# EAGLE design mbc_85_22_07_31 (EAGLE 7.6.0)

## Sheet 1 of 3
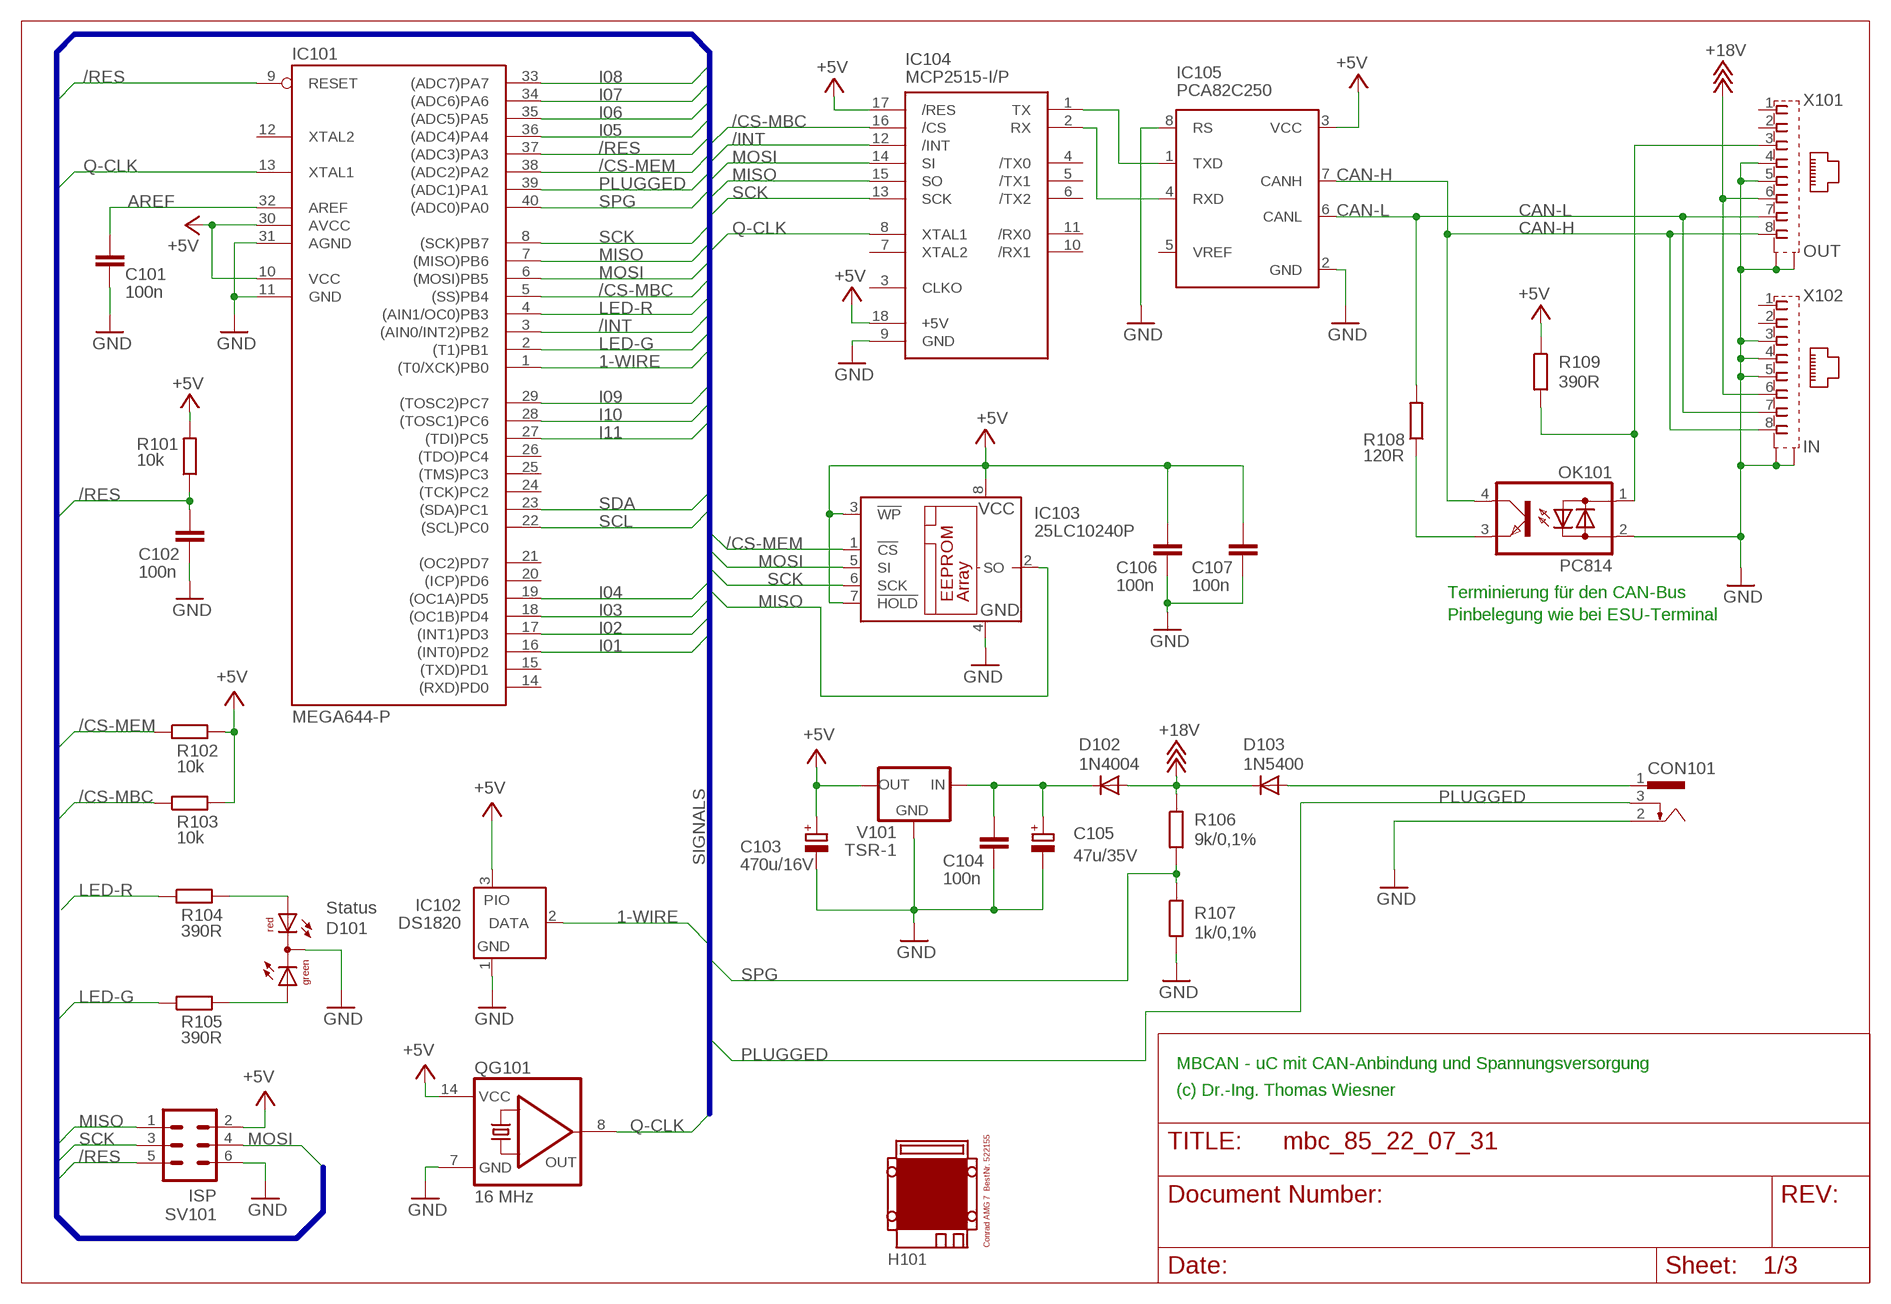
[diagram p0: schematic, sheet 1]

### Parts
C101  100n  C-EU025-025X050  [C025-025X050]
C102  100n  C-EU025-025X050  [C025-025X050]
C103  470u/16V  CPOL-EUE3.5-8  [E3,5-8]
C104  100n  C-EU025-025X050  [C025-025X050]
C105  47u/35V  CPOL-EUE2.5-7  [E2,5-7]
C106  100n  C-EU025-025X050  [C025-025X050]
C107  100n  C-EU025-025X050  [C025-025X050]
CON101  POWER-JACK  [POWER-JACK]
D101  Status  DUOLED5MM  [DUOLED5MM]
D102  1N4004  [DO41-10]
D103  1N5400  [DO201-15]
H101  MODULGEHÄUSE-AMG-7  [MODULGEHÄUSE-AMG-7]
IC101  MEGA644-P  MEGA323-P  [DIL40]
IC102  DS1820  DS2405  [TO92-]
IC103  25LC10240P  25LC040P  [DIL8]
IC104  MCP2515-I/P  MCP2510-I/P  [DIL18]
IC105  PCA82C250  [DIL08]
OK101  PC814  [DIL04]
QG101  16 MHz  QG5860  [DIL14S]
R101  10k  R-EU_0207/10  [0207/10]
R102  10k  R-EU_0207/10  [0207/10]
R103  10k  R-EU_0207/10  [0207/10]
R104  390R  R-EU_0207/10  [0207/10]
R105  390R  R-EU_0207/10  [0207/10]
R106  9k/0,1%  R-EU_0207/10  [0207/10]
R107  1k/0,1%  R-EU_0207/10  [0207/10]
R108  120R  R-EU_0207/10  [0207/10]
R109  390R  R-EU_0207/10  [0207/10]
SV101  ISP  ML6  [ML6]
V101  TSR-1  [TRACO-TSR-1]
X101  OUT  0446200002  [0446200002]
X102  IN  0446200002  [0446200002]

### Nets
1-WIRE: IC101.1((T0/XCK)PB0) IC102.2(DATA)
+5V: C103.+ C106.1 C107.1 IC101.10(VCC) IC101.30(AVCC) IC102.3(PIO) IC103.3(!WP) IC103.7(!HOLD) IC103.8(VCC) IC104.17(/RES) IC104.18(+5V) IC105.3(VCC) QG101.14(VCC) R101.2 R102.2 R103.2 R109.1 SV101.2 V101.OUT ; also sheet 2
+18V: D102.A D103.C R106.1 X101.6 X102.6
/CS-MBC: IC101.5((SS)PB4) IC104.16(/CS) R103.1
/CS-MEM: IC101.38((ADC2)PA2) IC103.1(!CS) R102.1
/INT: IC101.3((AIN0/INT2)PB2) IC104.12(/INT)
/RES: C102.1 IC101.9(RESET) IC101.37((ADC3)PA3) R101.1 SV101.5
AREF: C101.1 IC101.32(AREF)
CAN-H: IC105.7(CANH) OK101.4(C) X101.8 X102.8
CAN-L: IC105.6(CANL) R108.2 X101.7 X102.7
GND: C101.2 C102.2 C103.- C104.2 C105.- C106.2 C107.2 CON101.2 D101.K(C) IC101.11(GND) IC101.31(AGND) IC102.1(GND) IC103.4(GND) IC104.9(GND) IC105.2(GND) IC105.8(RS) OK101.2(AC2) QG101.7(GND) R107.2 SV101.6 V101.GND X101.4 X101.5 X101.S@1(S1) X101.S@2(S2) X102.3 X102.4 X102.5 X102.S@1(S1) X102.S@2(S2) ; also sheet 2
I01: IC101.16((INT0)PD2) ; also sheet 2
I02: IC101.17((INT1)PD3) ; also sheet 2
I03: IC101.18((OC1B)PD4) ; also sheet 2
I04: IC101.19((OC1A)PD5) ; also sheet 2
I05: IC101.36((ADC4)PA4) ; also sheet 2
I06: IC101.35((ADC5)PA5) ; also sheet 2
I07: IC101.34((ADC6)PA6) ; also sheet 2
I08: IC101.33((ADC7)PA7) ; also sheet 2
I09: IC101.29((TOSC2)PC7) ; also sheet 2
I10: IC101.28((TOSC1)PC6) ; also sheet 2
I11: IC101.27((TDI)PC5) ; also sheet 2
LED-G: IC101.2((T1)PB1) R105.1
LED-R: IC101.4((AIN1/OC0)PB3) R104.1
MISO: IC101.7((MISO)PB6) IC103.2(SO) IC104.15(SO) SV101.1
MOSI: IC101.6((MOSI)PB5) IC103.5(SI) IC104.14(SI) SV101.4
N$1: IC104.1(TX) IC105.1(TXD)
N$2: IC104.2(RX) IC105.4(RXD)
N$4: OK101.3(E) R108.1
N$6: C104.1 C105.+ D102.C V101.IN
N$7: OK101.1(AC1) R109.2 X101.3
N$9: D101.AR R104.2
N$13: D101.AG R105.2
PLUGGED: CON101.3 IC101.39((ADC1)PA1)
Q-CLK: IC101.13(XTAL1) IC104.8(XTAL1) QG101.8(OUT)
SCK: IC101.8((SCK)PB7) IC103.6(SCK) IC104.13(SCK) SV101.3
SCL: IC101.22((SCL)PC0) ; also sheet 2
SDA: IC101.23((SDA)PC1) ; also sheet 2
SPG: IC101.40((ADC0)PA0) R106.2 R107.1
V-NETZTEIL1: CON101.1 D103.A
Unconnected: IC101.12(XTAL2) IC101.14((RXD)PD0) IC101.15((TXD)PD1) IC101.20((ICP)PD6) IC101.21((OC2)PD7) IC101.24((TCK)PC2) IC101.25((TMS)PC3) IC101.26((TDO)PC4) IC104.3(CLKO) IC104.4(/TX0) IC104.5(/TX1) IC104.6(/TX2) IC104.7(XTAL2) IC104.10(/RX1) IC104.11(/RX0) IC105.5(VREF) X101.1 X101.2 X102.1 X102.2

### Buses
SIGNALS

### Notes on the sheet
- Terminierung für den CAN-Bus
- Pinbelegung wie bei ESU-Terminal
- MBCAN - uC mit CAN-Anbindung und Spannungsversorgung
- (c) Dr.-Ing. Thomas Wiesner

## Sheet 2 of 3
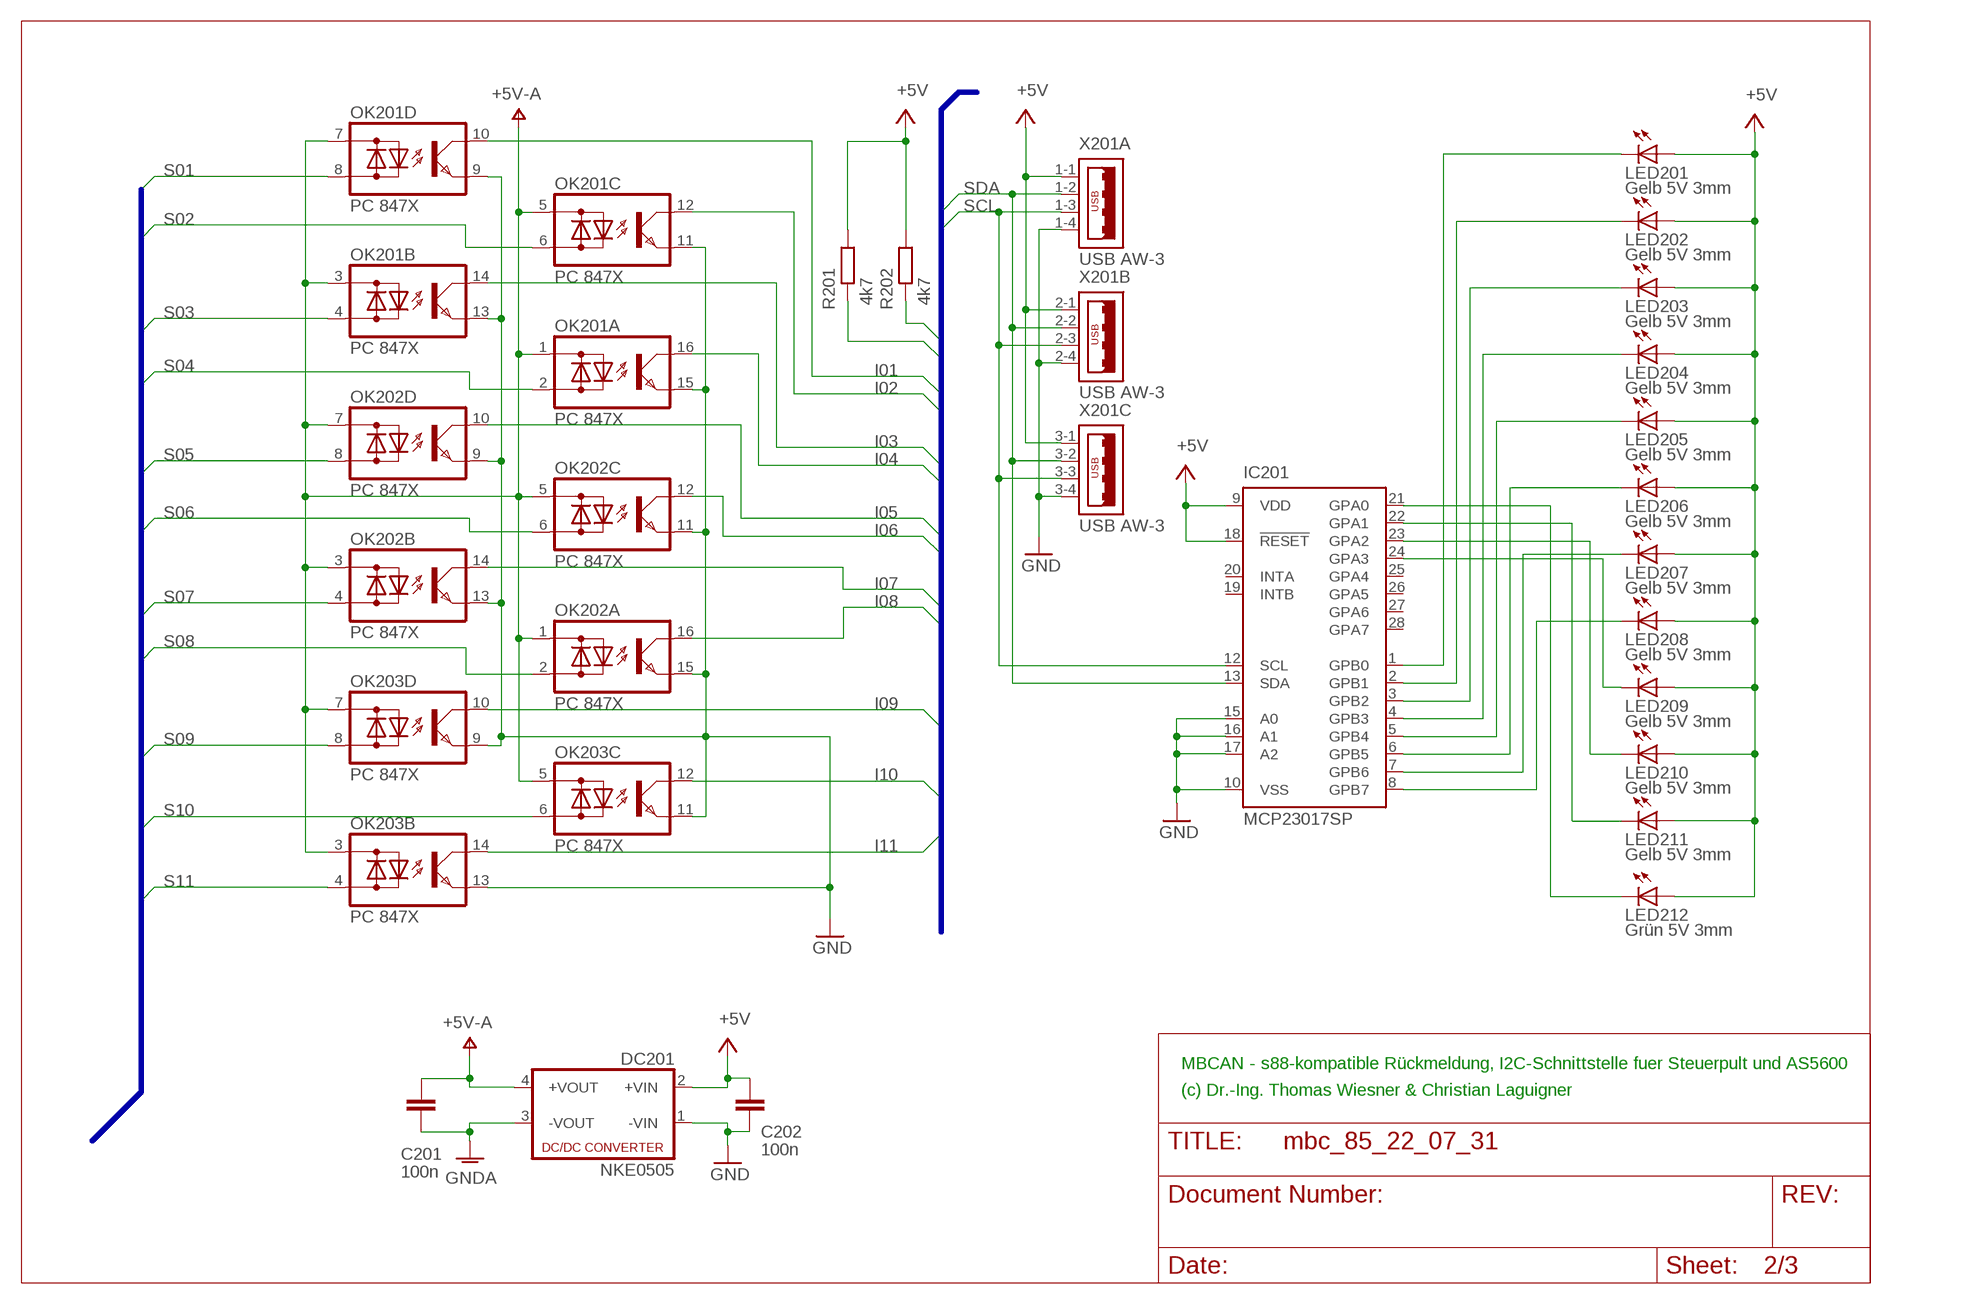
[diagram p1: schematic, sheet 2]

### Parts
C201  100n  C-EU025-025X050  [C025-025X050]
C202  100n  C-EU025-025X050  [C025-025X050]
DC201  NKE0505  NME  [NME]
IC201  MCP23017SP  [DIL28-3]
LED201  Gelb 5V 3mm  LED3MM  [LED3MM]
LED202  Gelb 5V 3mm  LED3MM  [LED3MM]
LED203  Gelb 5V 3mm  LED3MM  [LED3MM]
LED204  Gelb 5V 3mm  LED3MM  [LED3MM]
LED205  Gelb 5V 3mm  LED3MM  [LED3MM]
LED206  Gelb 5V 3mm  LED3MM  [LED3MM]
LED207  Gelb 5V 3mm  LED3MM  [LED3MM]
LED208  Gelb 5V 3mm  LED3MM  [LED3MM]
LED209  Gelb 5V 3mm  LED3MM  [LED3MM]
LED210  Gelb 5V 3mm  LED3MM  [LED3MM]
LED211  Gelb 5V 3mm  LED3MM  [LED3MM]
LED212  Grün 5V 3mm  LED3MM  [LED3MM]
OK201  PC 847X  TIL196  [DIL16]
OK202  PC 847X  TIL196  [DIL16]
OK203  PC 847X  TIL196  [DIL16]
R201  4k7  R-EU_0207/10  [0207/10]
R202  4k7  R-EU_0207/10  [0207/10]
X201  USB AW-3  USB_3P-85-32003-00X-1  [85-32003-00X-1]

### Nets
+5V: C202.1 DC201.2(+VIN) IC201.9(VDD) IC201.18(!RESET) LED201.A LED202.A LED203.A LED204.A LED205.A LED206.A LED207.A LED208.A LED209.A LED210.A LED211.A LED212.A R201.2 R202.2 X201.1-1 X201.2-1 X201.3-1 ; also sheet 1
GND: C202.2 DC201.1(-VIN) IC201.10(VSS) IC201.15(A0) IC201.16(A1) IC201.17(A2) OK201.9(D:E) OK201.11(C:E) OK201.13(B:E) OK201.15(A:E) OK202.9(D:E) OK202.11(C:E) OK202.13(B:E) OK202.15(A:E) OK203.9(D:E) OK203.11(C:E) OK203.13(B:E) X201.1-4 X201.2-4 X201.3-4 ; also sheet 1
GNDA: C201.2 DC201.3(-VOUT) ; also sheet 3
I01: OK201.10(D:C) ; also sheet 1
I02: OK201.12(C:C) ; also sheet 1
I03: OK201.14(B:C) ; also sheet 1
I04: OK201.16(A:C) ; also sheet 1
I05: OK202.10(D:C) ; also sheet 1
I06: OK202.12(C:C) ; also sheet 1
I07: OK202.14(B:C) ; also sheet 1
I08: OK202.16(A:C) ; also sheet 1
I09: OK203.10(D:C) ; also sheet 1
I10: OK203.12(C:C) ; also sheet 1
I11: OK203.14(B:C) ; also sheet 1
N$10: IC201.1(GPB0) LED201.K(C)
N$11: IC201.24(GPA3) LED209.K(C)
N$16: IC201.21(GPA0) LED212.K(C)
N$18: IC201.2(GPB1) LED202.K(C)
N$19: IC201.3(GPB2) LED203.K(C)
N$22: IC201.4(GPB3) LED204.K(C)
N$23: IC201.5(GPB4) LED205.K(C)
N$32: IC201.6(GPB5) LED206.K(C)
N$34: IC201.7(GPB6) LED207.K(C)
N$35: IC201.8(GPB7) LED208.K(C)
N$36: IC201.22(GPA1) LED211.K(C)
N$37: IC201.23(GPA2) LED210.K(C)
S01: OK201.8(D:AC2) ; also sheet 3
S02: OK201.6(C:AC2) ; also sheet 3
S03: OK201.4(B:AC2) ; also sheet 3
S04: OK201.2(A:AC2) ; also sheet 3
S05: OK202.8(D:AC2) ; also sheet 3
S06: OK202.6(C:AC2) ; also sheet 3
S07: OK202.4(B:AC2) ; also sheet 3
S08: OK202.2(A:AC2) ; also sheet 3
S09: OK203.8(D:AC2) ; also sheet 3
S10: OK203.6(C:AC2) ; also sheet 3
S11: OK203.4(B:AC2) ; also sheet 3
SCL: IC201.12(SCL) R201.1 X201.1-3 X201.2-3 X201.3-3 ; also sheet 1
SDA: IC201.13(SDA) R202.1 X201.1-2 X201.2-2 X201.3-2 ; also sheet 1
V+: C201.1 DC201.4(+VOUT) OK201.1(A:AC1) OK201.3(B:AC1) OK201.5(C:AC1) OK201.7(D:AC1) OK202.1(A:AC1) OK202.3(B:AC1) OK202.5(C:AC1) OK202.7(D:AC1) OK203.3(B:AC1) OK203.5(C:AC1) OK203.7(D:AC1) ; supply symbol labelled +5V-A
Unconnected: IC201.19(INTB) IC201.20(INTA) IC201.25(GPA4) IC201.26(GPA5) IC201.27(GPA6) IC201.28(GPA7) OK203.1(A:AC1) OK203.2(A:AC2) OK203.15(A:E) OK203.16(A:C)

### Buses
B$1
B$2

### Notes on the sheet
- MBCAN - s88-kompatible Rückmeldung, I2C-Schnittstelle fuer Steuerpult und AS5600
- (c) Dr.-Ing. Thomas Wiesner & Christian Laguigner

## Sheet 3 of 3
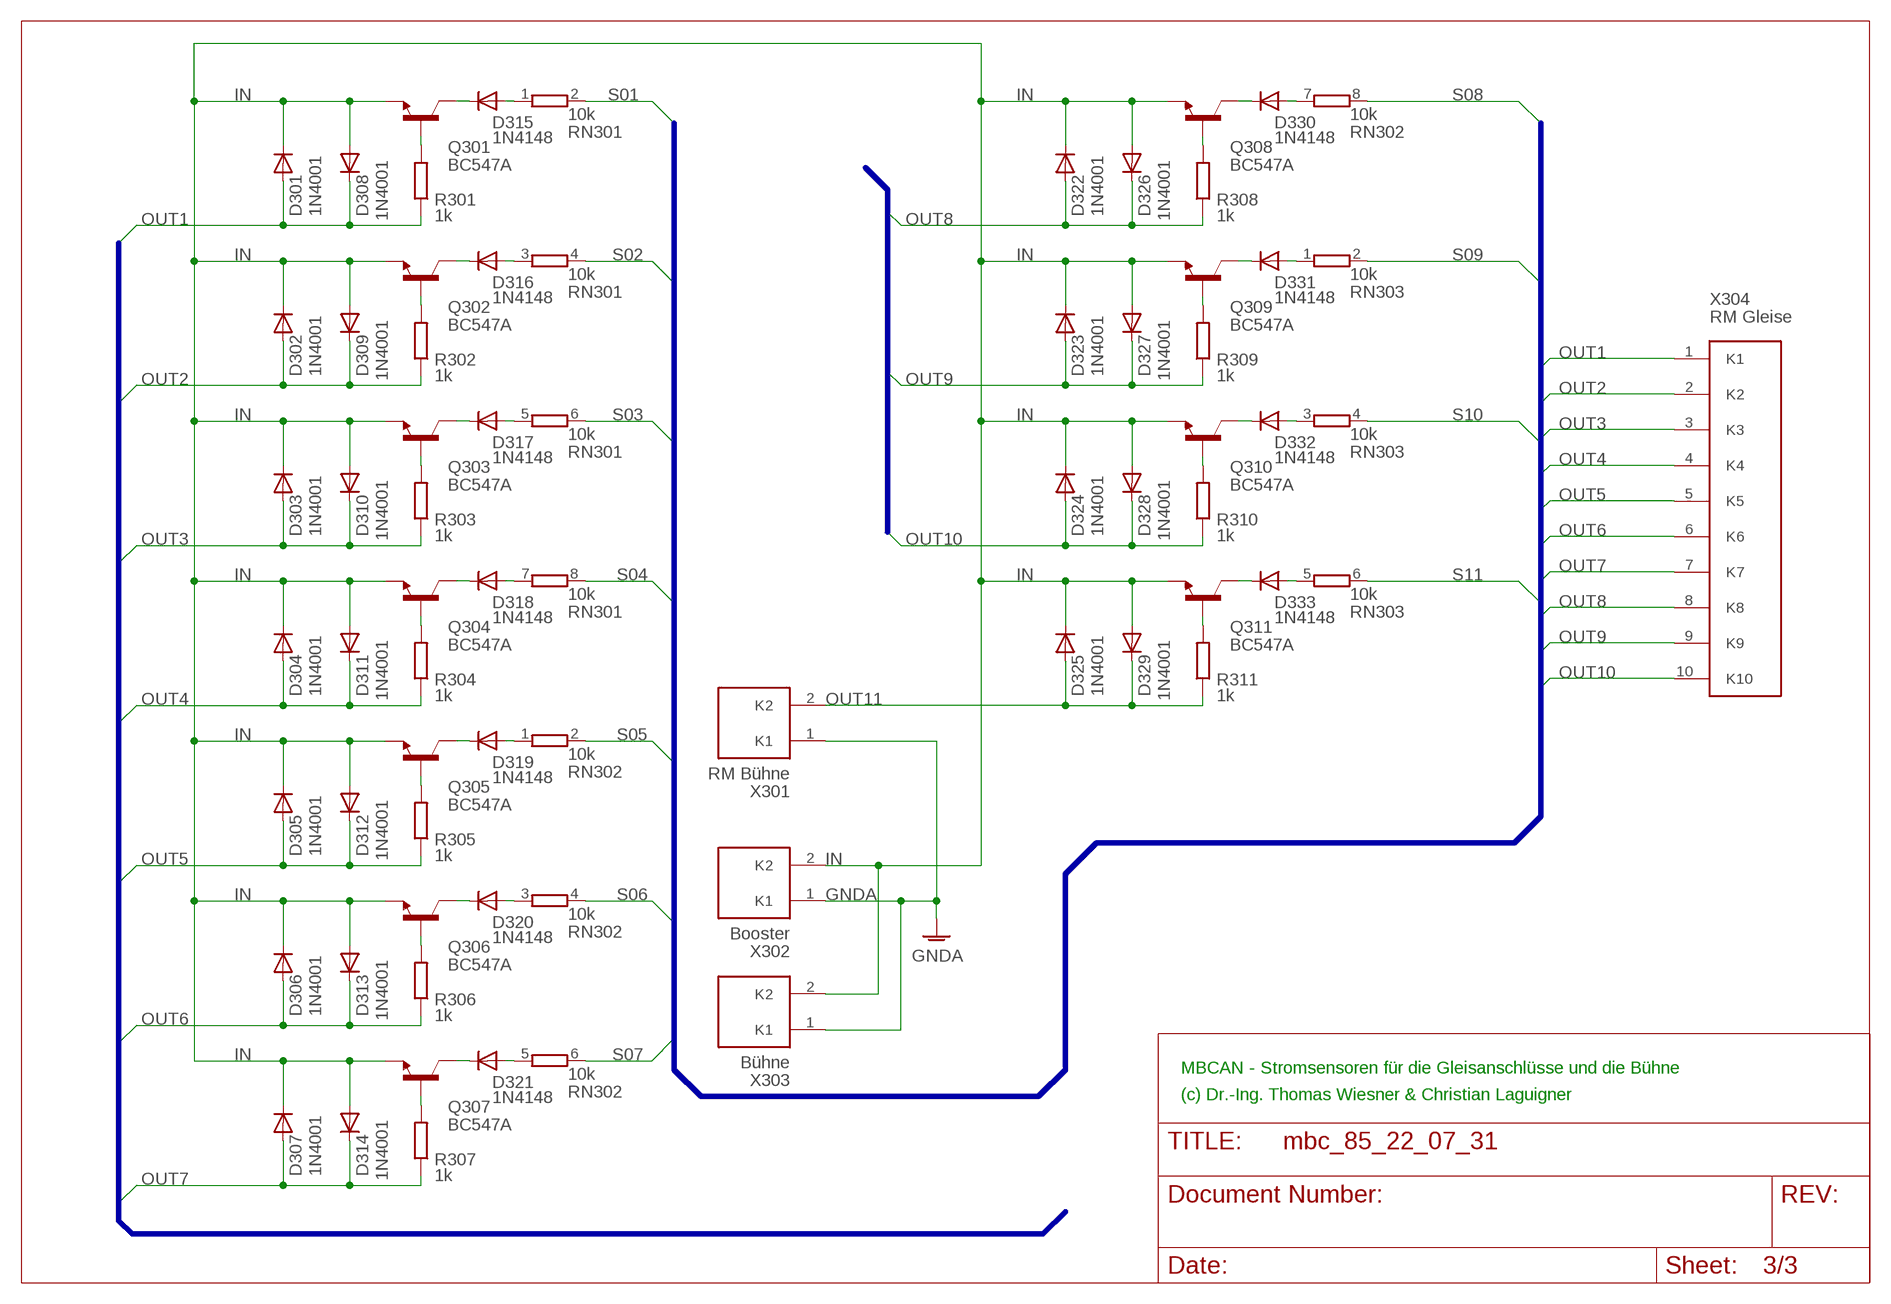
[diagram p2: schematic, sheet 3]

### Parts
D301  1N4001  1N4004  [DO41-10]
D302  1N4001  1N4004  [DO41-10]
D303  1N4001  1N4004  [DO41-10]
D304  1N4001  1N4004  [DO41-10]
D305  1N4001  1N4004  [DO41-10]
D306  1N4001  1N4004  [DO41-10]
D307  1N4001  1N4004  [DO41-10]
D308  1N4001  1N4004  [DO41-10]
D309  1N4001  1N4004  [DO41-10]
D310  1N4001  1N4004  [DO41-10]
D311  1N4001  1N4004  [DO41-10]
D312  1N4001  1N4004  [DO41-10]
D313  1N4001  1N4004  [DO41-10]
D314  1N4001  1N4004  [DO41-10]
D315  1N4148  1N4148DO35-10  [DO35-10]
D316  1N4148  1N4148DO35-10  [DO35-10]
D317  1N4148  1N4148DO35-10  [DO35-10]
D318  1N4148  1N4148DO35-10  [DO35-10]
D319  1N4148  1N4148DO35-10  [DO35-10]
D320  1N4148  1N4148DO35-10  [DO35-10]
D321  1N4148  1N4148DO35-10  [DO35-10]
D322  1N4001  1N4004  [DO41-10]
D323  1N4001  1N4004  [DO41-10]
D324  1N4001  1N4004  [DO41-10]
D325  1N4001  1N4004  [DO41-10]
D326  1N4001  1N4004  [DO41-10]
D327  1N4001  1N4004  [DO41-10]
D328  1N4001  1N4004  [DO41-10]
D329  1N4001  1N4004  [DO41-10]
D330  1N4148  1N4148DO35-10  [DO35-10]
D331  1N4148  1N4148DO35-10  [DO35-10]
D332  1N4148  1N4148DO35-10  [DO35-10]
D333  1N4148  1N4148DO35-10  [DO35-10]
Q301  BC547A  [TO92]
Q302  BC547A  [TO92]
Q303  BC547A  [TO92]
Q304  BC547A  [TO92]
Q305  BC547A  [TO92]
Q306  BC547A  [TO92]
Q307  BC547A  [TO92]
Q308  BC547A  [TO92]
Q309  BC547A  [TO92]
Q310  BC547A  [TO92]
Q311  BC547A  [TO92]
R301  1k  R-EU_0207/10  [0207/10]
R302  1k  R-EU_0207/10  [0207/10]
R303  1k  R-EU_0207/10  [0207/10]
R304  1k  R-EU_0207/10  [0207/10]
R305  1k  R-EU_0207/10  [0207/10]
R306  1k  R-EU_0207/10  [0207/10]
R307  1k  R-EU_0207/10  [0207/10]
R308  1k  R-EU_0207/10  [0207/10]
R309  1k  R-EU_0207/10  [0207/10]
R310  1k  R-EU_0207/10  [0207/10]
R311  1k  R-EU_0207/10  [0207/10]
RN301  10k  E4RP  [SIL8]
RN302  10k  E4RP  [SIL8]
RN303  10k  E4RP  [SIL8]
X301  RM Bühne  AKL182-2  [AKL182-2]
X302  Booster  AKL182-2  [AKL182-2]
X303  Bühne  AKL182-2  [AKL182-2]
X304  RM Gleise  AKL182-10  [AKL182-10]

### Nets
GNDA: X301.1(K1) X302.1(K1) X303.1(K1) ; also sheet 2
IN: D301.C D302.C D303.C D304.C D305.C D306.C D307.C D308.A D309.A D310.A D311.A D312.A D313.A D314.A D322.C D323.C D324.C D325.C D326.A D327.A D328.A D329.A Q301.1(E) Q302.1(E) Q303.1(E) Q304.1(E) Q305.1(E) Q306.1(E) Q307.1(E) Q308.1(E) Q309.1(E) Q310.1(E) Q311.1(E) X302.2(K2) X303.2(K2)
N$27: Q301.2(B) R301.2
N$33: D315.C Q301.3(C)
N$38: D315.A RN301.1
N$40: Q302.2(B) R302.2
N$41: D316.C Q302.3(C)
N$49: D316.A RN301.3
N$51: Q303.2(B) R303.2
N$52: D317.C Q303.3(C)
N$53: D317.A RN301.5
N$55: Q304.2(B) R304.2
N$56: D318.C Q304.3(C)
N$57: D318.A RN301.7
N$59: Q305.2(B) R305.2
N$60: D319.C Q305.3(C)
N$61: D319.A RN302.1
N$63: Q306.2(B) R306.2
N$66: D320.C Q306.3(C)
N$67: D320.A RN302.3
N$69: Q307.2(B) R307.2
N$70: D321.C Q307.3(C)
N$71: D321.A RN302.5
N$73: Q308.2(B) R308.2
N$74: D330.C Q308.3(C)
N$75: D330.A RN302.7
N$77: Q309.2(B) R309.2
N$78: D331.C Q309.3(C)
N$79: D331.A RN303.1
N$81: Q310.2(B) R310.2
N$82: D332.C Q310.3(C)
N$83: D332.A RN303.3
N$85: Q311.2(B) R311.2
N$86: D333.C Q311.3(C)
N$87: D333.A RN303.5
OUT1: D301.A D308.C R301.1 X304.1(K1)
OUT2: D302.A D309.C R302.1 X304.2(K2)
OUT3: D303.A D310.C R303.1 X304.3(K3)
OUT4: D304.A D311.C R304.1 X304.4(K4)
OUT5: D305.A D312.C R305.1 X304.5(K5)
OUT6: D306.A D313.C R306.1 X304.6(K6)
OUT7: D307.A D314.C R307.1 X304.7(K7)
OUT8: D322.A D326.C R308.1 X304.8(K8)
OUT9: D323.A D327.C R309.1 X304.9(K9)
OUT10: D324.A D328.C R310.1 X304.10(K10)
OUT11: D325.A D329.C R311.1 X301.2(K2)
S01: RN301.2 ; also sheet 2
S02: RN301.4 ; also sheet 2
S03: RN301.6 ; also sheet 2
S04: RN301.8 ; also sheet 2
S05: RN302.2 ; also sheet 2
S06: RN302.4 ; also sheet 2
S07: RN302.6 ; also sheet 2
S08: RN302.8 ; also sheet 2
S09: RN303.2 ; also sheet 2
S10: RN303.4 ; also sheet 2
S11: RN303.6 ; also sheet 2
Unconnected: RN303.7 RN303.8

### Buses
B$3
B$4
B$5

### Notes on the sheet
- MBCAN - Stromsensoren für die Gleisanschlüsse und die Bühne
- (c) Dr.-Ing. Thomas Wiesner & Christian Laguigner

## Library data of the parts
C101 C102 C104 C106 C107 C201 C202 = rcl:C-EU: CAPACITOR, European symbol
C103 C105 = rcl:CPOL-EU: POLARIZED CAPACITOR, European symbol
CON101 = mbc:POWER-JACK: Power-Stecker für 2,5 mm Hohlbuchse
D101 = led:DUOLED5MM: DUO LED 2 colors, 5 mm, round
D102 D301-D314 D322-D329 = diode:1N4004: DIODE
D103 = diode:1N5400: DIODE
D315-D321 D330-D333 = diode:1N4148: DIODE
DC201 = dc-dc-converter:NME: DC-DC CONVERTER; MF: C & D TECHNOLOGIES, INC; MPN: NME1205D; OC_FARNELL: 1021466; OC_NEWARK: 98B8198
H101 = mbc:MODULGEHÄUSE-AMG-7: Gehäuse
IC101 = atmel:MEGA323-P: MICROCONTROLLER 32 Kbytes FLASH 2 Kbytes SRAM 1 Kbytes EEPROM USART 8-channel 10 bit ADC Source: avr.lbr; OC_FARNELL: unknown; OC_NEWARK: unknown
IC102 = maxim:DS2405: Addressable Switch DALLAS Semiconductor; MF: DALLAS SEMICONDUCTOR; MPN: DS2405; OC_FARNELL: 1188025; OC_NEWARK: 06F4645
IC103 = microchip:25*: Serial EEPROM 4K/ 8K , SPI bus; MF: MICROCHIP; MPN: 25LC040/P; OC_FARNELL: 9758100; OC_NEWARK: 96K4091
IC104 = mbc:MCP2510: BASIC-CAN 2.0a Controller Stand-alone CAN controller von Microchip
IC105 = micro-philips:PCA82C250: CAN CONTROLLER INTERFACE; OC_FARNELL: 3692358; OC_NEWARK: unknown
IC201 = microchip:MCP23017: http://ww1.microchip.com/downloads/en/DeviceDoc/21952a.pdf Source: http://ww1.microchip.com/downloads/en/DeviceDoc/21952a.pdf; MF: MICROCHIP; MPN: MCP23017-E/SP; OC_FARNELL: 1332088; OC_NEWARK: 31K2959
LED201-LED212 = led:LED: LED
OK101 = optocoupler:PC814: SHARP OPTO COUPLER; OC_FARNELL: 9707662; OC_NEWARK: unknown
OK201-OK203 = optocoupler:TIL196: TEXAS INSTRUMENTS OPTO COUPLER; MPN: TIL 196; OC_FARNELL: 1683367; OC_NEWARK: 05R6476
Q301-Q311 = transistor-npn:BC547*: NPN Transistor
QG101 = crystal:QG5860: CRYSTAL RESONATOR; OC_FARNELL: unknown; OC_NEWARK: unknown
R101-R109 R201 R202 R301-R311 = resistor:R-EU_: RESISTOR, European symbol
RN301-RN303 = resistor-sil:E4RP: SIL RESISTOR; OC_FARNELL: unknown; OC_NEWARK: unknown
SV101 = con-ml:ML6: HARTING; OC_FARNELL: unknown; OC_NEWARK: unknown
V101 = mbc:TSR-1: Spannungsregler Hersteller: TRACO Typ: TSR-1 5V: TSR 1-2450 Spg: 5V Strom: 1A Reichelt TSR 1-2450
X101 X102 = mbc:0446200002: RJ-45 INVERTED MODULAR JACK ASSEMBLY WITH RJ-11 KEEPOUT FEATURE Source: Data sheet MOLEX 0446200002 BUCHSE, RJ45, GESCHIRMT Source: Farnell; MF: MOLEX; MPN: 0446200002; OC_FARNELL: 9251910
X201 = con-cypressindustries:USB_3P-: Triple USB Connector Source: www.cypressindustries.com; OC_FARNELL: unknown; OC_NEWARK: unknown
X301-X303 = mbc:AKL182-2: Steckverbinder
X304 = mbc:AKL182-10: Steckverbinder Rastermaß: 3,5 mm Hersteller: RIA Reichelt: Bestellnummer AKL 182-10

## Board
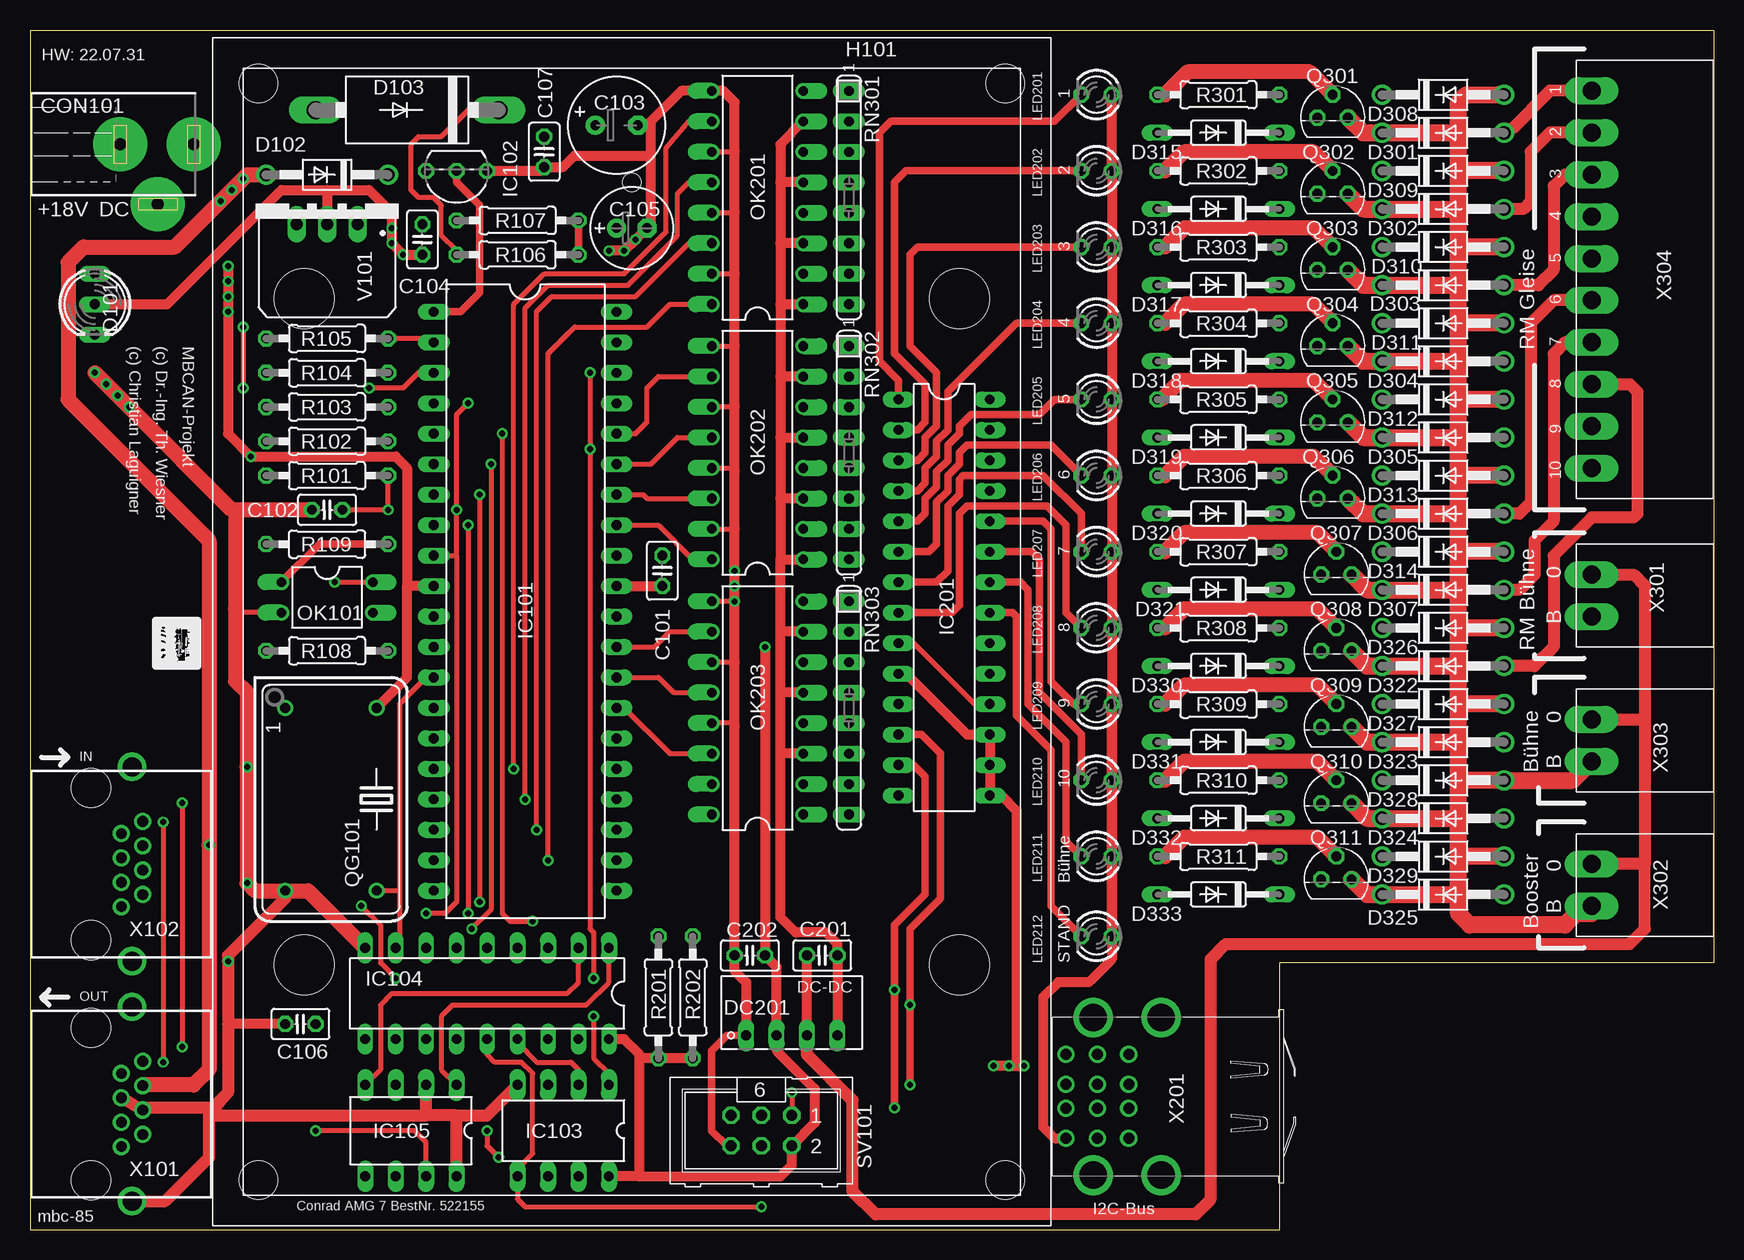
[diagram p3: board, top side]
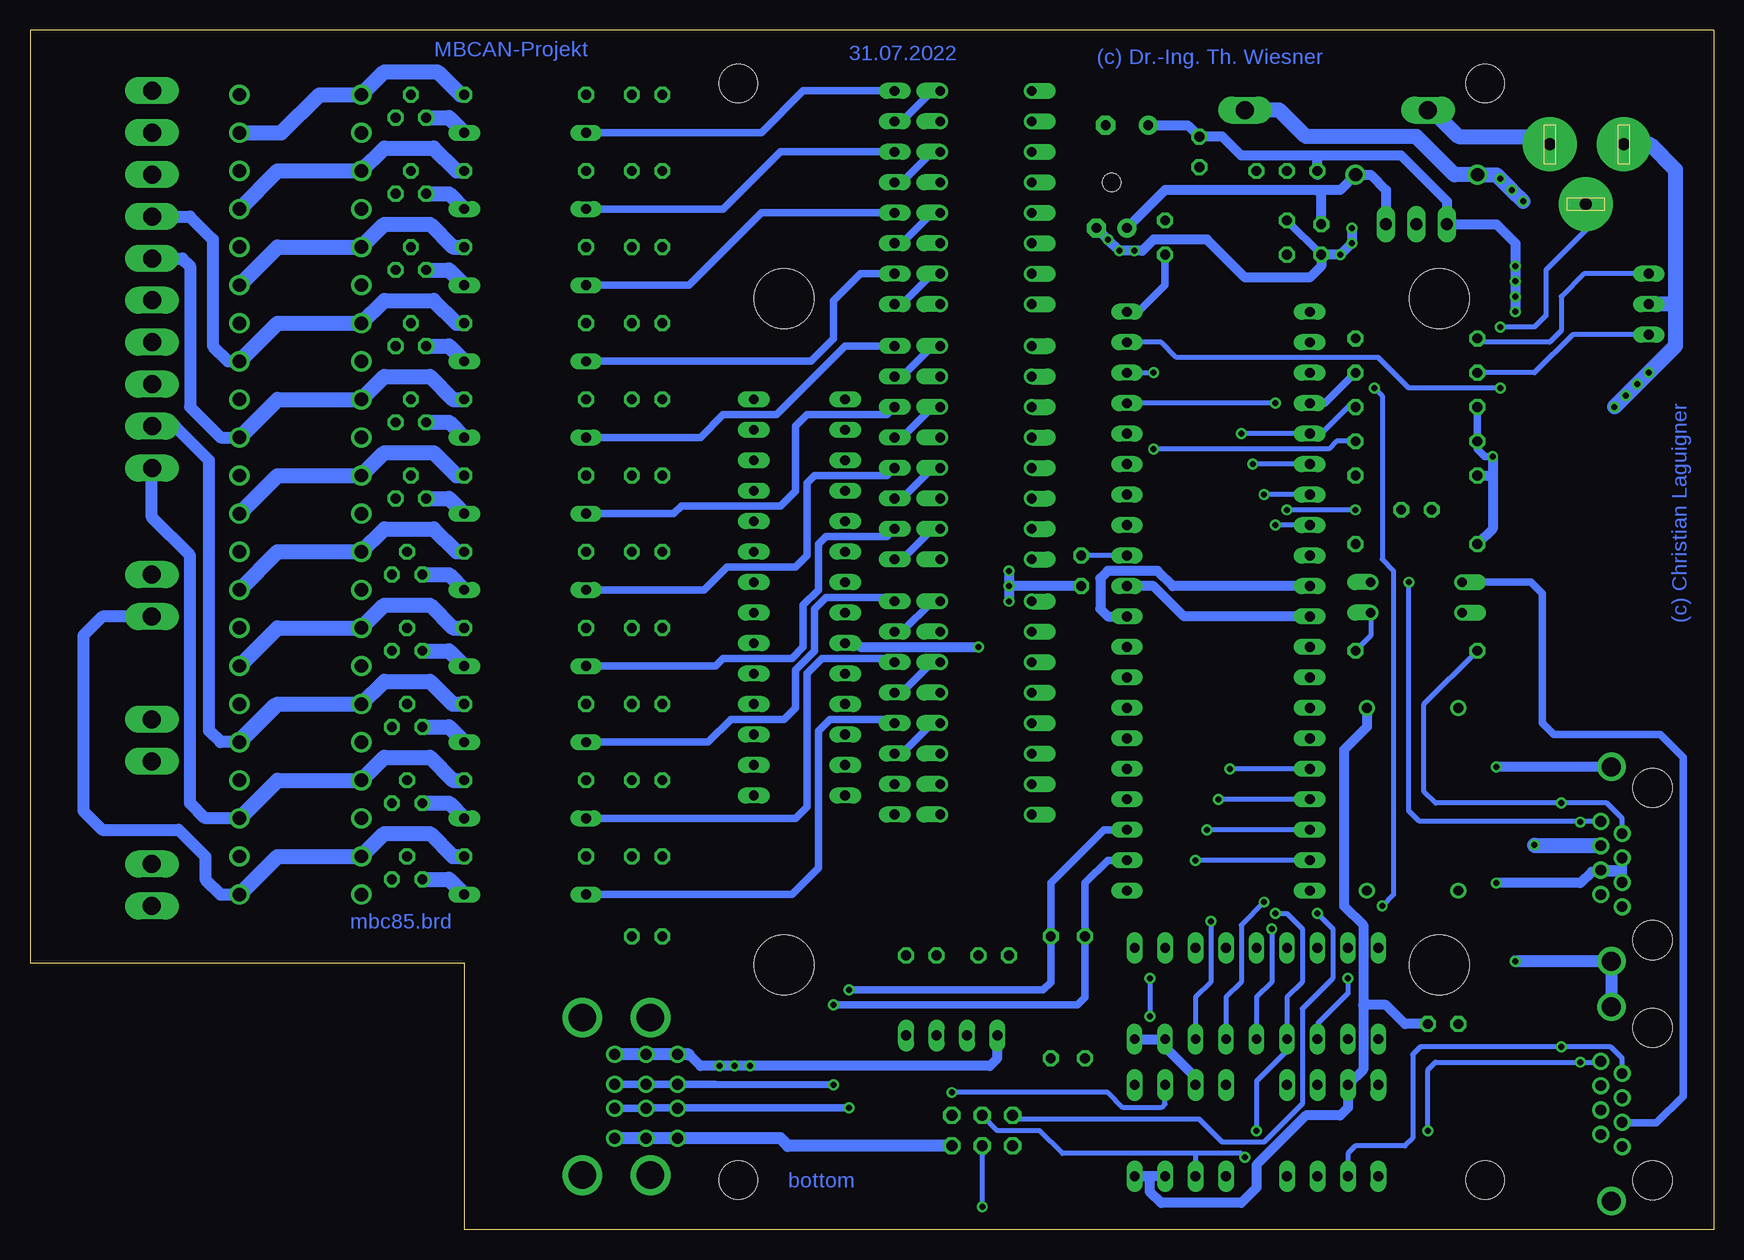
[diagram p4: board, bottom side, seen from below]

Size 140.34 x 100.01 mm. Coordinates in mm from the lower left corner, seen from the top.
Outline: 0,0.02 0,100.01 140.34,100.01 140.34,22.23 104.14,22.23 104.14,0 0,0
Copper layers (1*16): Top 0.035mm / dielectric 1.5mm / Bottom 0.035mm
Design rules "default *": minimum track width 10mil, minimum drill 0.5mm, track to track 8mil, track to pad 8mil, pad to pad 8mil, via to via 8mil, smd to smd 8mil, copper to edge 40mil, drill to drill 8mil, minimum pad ring 10mil, minimum via ring 8mil, stop-mask expansion 4mil, vias tented up to drill 0mil, thermal gap 10mil

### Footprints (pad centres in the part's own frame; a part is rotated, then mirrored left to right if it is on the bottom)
C025-025X050 = drill 0.813 octagon: 1 -1.27,0; 2 1.27,0
E3,5-8 = drill 0.813 pad 1.6: + -1.778,0 | drill 0.813 pad 1.6 octagon: - 1.778,0
E2,5-7 = drill 0.813 pad 1.6: + -1.27,0 | drill 0.813 pad 1.6 octagon: - 1.27,0
POWER-JACK = drill 1 pad 4.5: 1 0,6.03; 2 0,-0.12; 3 5,3.03
DUOLED5MM = drill 0.813 long: AG -2.54,0; AR 2.54,0; K 0,0
DO41-10 = drill 1.118: A 5.08,0; C -5.08,0
DO201-15 = drill 1.499 long: A 7.62,0; C -7.62,0
DO35-10 = drill 0.813 long: A 5.08,0; C -5.08,0
NME = drill 0.813 long: 1 0,3.81; 2 0,1.27; 3 0,-1.27; 4 0,-3.81
MODULGEHÄUSE-AMG-7 = hole 3.2: -45.72,-31.115; -45.72,31.115; 45.72,31.115; 45.72,-31.115 | hole 5: -27.781,-27.305; 27.781,-27.305; -27.781,27.305; 27.781,27.305 | hole 1.5: -37.465,0
DIL40 = drill 0.813 long: 1 -24.13,-7.62; 2 -21.59,-7.62; 3 -19.05,-7.62; 4 -16.51,-7.62; 5 -13.97,-7.62; 6 -11.43,-7.62; 7 -8.89,-7.62; 8 -6.35,-7.62; 9 -3.81,-7.62; 10 -1.27,-7.62; 11 1.27,-7.62; 12 3.81,-7.62; 13 6.35,-7.62; 14 8.89,-7.62; 15 11.43,-7.62; 16 13.97,-7.62; 17 16.51,-7.62; 18 19.05,-7.62; 19 21.59,-7.62; 20 24.13,-7.62; 21 24.13,7.62; 22 21.59,7.62; 23 19.05,7.62; 24 16.51,7.62; 25 13.97,7.62; 26 11.43,7.62; 27 8.89,7.62; 28 6.35,7.62; 29 3.81,7.62; 30 1.27,7.62; 31 -1.27,7.62; 32 -3.81,7.62; 33 -6.35,7.62; 34 -8.89,7.62; 35 -11.43,7.62; 36 -13.97,7.62; 37 -16.51,7.62; 38 -19.05,7.62; 39 -21.59,7.62; 40 -24.13,7.62
TO92- = drill 0.813 octagon: 1 -2.54,0; 2 0,0; 3 2.54,0
DIL8 = drill 0.813 long: 1 -3.81,-3.81; 2 -1.27,-3.81; 3 1.27,-3.81; 4 3.81,-3.81; 5 3.81,3.81; 6 1.27,3.81; 7 -1.27,3.81; 8 -3.81,3.81
DIL18 = drill 0.813 long: 1 -10.16,-3.81; 2 -7.62,-3.81; 3 -5.08,-3.81; 4 -2.54,-3.81 | drill 0.8 long: 5 0,-3.81; 6 2.54,-3.81; 7 5.08,-3.81; 8 7.62,-3.81; 9 10.16,-3.81; 10 10.16,3.81; 11 7.62,3.81; 12 5.08,3.81; 13 2.54,3.81; 14 0,3.81; 15 -2.54,3.81; 16 -5.08,3.81; 17 -7.62,3.81; 18 -10.16,3.81
DIL08 = drill 0.813 long: 1 -3.81,-3.81; 2 -1.27,-3.81; 3 1.27,-3.81; 4 3.81,-3.81; 5 3.81,3.81; 6 1.27,3.81; 7 -1.27,3.81; 8 -3.81,3.81
DIL28-3 = drill 0.813 long: 1 -16.51,-3.81; 2 -13.97,-3.81; 3 -11.43,-3.81; 4 -8.89,-3.81; 5 -6.35,-3.81; 6 -3.81,-3.81; 7 -1.27,-3.81; 8 1.27,-3.81; 9 3.81,-3.81; 10 6.35,-3.81; 11 8.89,-3.81; 12 11.43,-3.81; 13 13.97,-3.81; 14 16.51,-3.81; 15 16.51,3.81; 16 13.97,3.81; 17 11.43,3.81; 18 8.89,3.81; 19 6.35,3.81; 20 3.81,3.81; 21 1.27,3.81; 22 -1.27,3.81; 23 -3.81,3.81; 24 -6.35,3.81; 25 -8.89,3.81; 26 -11.43,3.81; 27 -13.97,3.81; 28 -16.51,3.81
LED3MM = drill 0.813 octagon: A -1.27,0; K 1.27,0
DIL04 = drill 0.813 offset: 1 -1.27,-3.81; 2 1.27,-3.81; 3 1.27,3.81; 4 -1.27,3.81
DIL16 = drill 0.813 offset: 1 -8.89,-3.81; 2 -6.35,-3.81; 3 -3.81,-3.81; 4 -1.27,-3.81; 5 1.27,-3.81; 6 3.81,-3.81; 7 6.35,-3.81; 8 8.89,-3.81; 9 8.89,3.81; 10 6.35,3.81; 11 3.81,3.81; 12 1.27,3.81; 13 -1.27,3.81; 14 -3.81,3.81; 15 -6.35,3.81; 16 -8.89,3.81
TO92 = drill 0.813 octagon: 1 1.27,0; 2 0,1.905; 3 -1.27,0
DIL14S = drill 0.813: 1 -7.62,-3.81; 7 7.62,-3.81; 8 7.62,3.81; 14 -7.62,3.81
0207/10 = drill 0.813 octagon: 1 -5.08,0; 2 5.08,0
SIL8 = drill 0.813 long: 1 -8.89,0; 2 -6.35,0; 3 -3.81,0; 4 -1.27,0; 5 1.27,0; 6 3.81,0; 7 6.35,0; 8 8.89,0
ML6 = drill 0.914 octagon: 1 -2.54,-1.27; 2 -2.54,1.27; 3 0,-1.27; 4 0,1.27; 5 2.54,-1.27; 6 2.54,1.27
TRACO-TSR-1 = drill 1.016 long: GND 0,2.54; IN -2.54,2.54; OUT 2.54,2.54
0446200002 = drill 0.889 pad 1.422: 1 3.556,2.54; 2 2.54,4.318; 3 1.524,2.54; 4 0.508,4.318; 5 -0.508,2.54; 6 -1.524,4.318; 7 -2.54,2.54; 8 -3.556,4.318 | drill 1.575 pad 2.286: S@1 -8.103,3.429; S@2 8.103,3.429 | hole 3.251: 6.35,0; -6.35,0
85-32003-00X-1 = drill 0.92 pad 1.27: 1-1 2.71,3.5; 1-2 2.71,1; 1-3 2.71,-1; 1-4 2.71,-3.5; 2-1 5.33,3.5; 2-2 5.33,1; 2-3 5.33,-1; 2-4 5.33,-3.5; 3-1 7.95,3.5; 3-2 7.95,1; 3-3 7.95,-1; 3-4 7.95,-3.5 | drill 2.3 pad 3: M1 0,6.57; M2 0,-6.57; M3 5.68,6.57; M4 5.68,-6.57
AKL182-2 = drill 1.5 pad 2.184 long: 1 0,1.587; 2 0,-1.913
AKL182-10 = drill 1.5 pad 2.184 long: 1 -3.5,15.58; 2 -3.5,12.08; 3 -3.5,8.58; 4 -3.5,5.088; 5 -3.5,1.595; 6 -3.5,-1.897; 7 -3.5,-5.397; 8 -3.5,-8.898; 9 -3.5,-12.398; 10 -3.5,-15.898

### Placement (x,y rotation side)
C101  52.7,54.93 270 top
C102  24.77,60.01 180 top
C103  48.9,92.08 0 top
C104  32.7,82.55 270 top
C105  50.16,83.5 0 top
C106  22.54,17.14 180 top
C107  42.86,89.85 270 top
C201  66.04,22.86 180 top
C202  60.01,22.86 180 top
CON101  7.62,90.49 270 top
D101  5.4,77.15 270 top
D102  24.77,87.95 180 top
D103  31.43,93.34 180 top
D301  117.79,91.44 0 top
D302  117.79,85.09 0 top
D303  117.79,78.74 0 top
D304  117.79,72.39 0 top
D305  117.79,66.04 0 top
D306  117.79,59.69 0 top
D307  117.79,53.34 0 top
D308  117.79,94.61 0 top
D309  117.79,88.27 0 top
D310  117.79,81.92 0 top
D311  117.79,75.56 0 top
D312  117.79,69.22 0 top
D313  117.79,62.87 0 top
D314  117.79,56.52 0 top
D315  99.06,91.44 180 top
D316  99.06,85.09 180 top
D317  99.06,78.74 180 top
D318  99.06,72.39 180 top
D319  99.06,66.04 180 top
D320  99.06,59.69 180 top
D321  99.06,53.34 180 top
D322  117.79,46.99 0 top
D323  117.79,40.64 0 top
D324  117.79,34.29 0 top
D325  117.79,27.94 0 top
D326  117.79,50.16 0 top
D327  117.79,43.81 0 top
D328  117.79,37.47 0 top
D329  117.79,31.11 0 top
D330  99.06,46.99 180 top
D331  99.06,40.64 180 top
D332  99.06,34.29 180 top
D333  99.06,27.94 180 top
DC201  63.5,16.19 90 top
H101  50.16,49.85 270 top
IC101  41.27,52.39 270 top
IC102  35.56,88.27 180 top
IC103  44.45,8.26 180 top
IC104  38.1,19.68 180 top
IC105  31.75,8.26 180 top
IC201  76.2,52.7 270 top
LED201  88.9,94.61 180 top
LED202  88.9,88.27 180 top
LED203  88.9,81.92 180 top
LED204  88.9,75.56 180 top
LED205  88.9,69.22 180 top
LED206  88.9,62.87 180 top
LED207  88.9,56.52 180 top
LED208  88.9,50.16 180 top
LED209  88.9,43.81 180 top
LED210  88.9,37.47 180 top
LED211  88.9,31.11 180 top
LED212  88.9,24.45 180 top
OK101  24.77,52.7 270 top
OK201  60.64,86.04 90 top
OK202  60.64,64.77 90 top
OK203  60.64,43.5 90 top
Q301  108.58,92.71 0 top
Q302  108.58,86.36 0 top
Q303  108.58,80.01 0 top
Q304  108.58,73.66 0 top
Q305  108.58,67.31 0 top
Q306  108.58,60.96 0 top
Q307  108.9,54.61 0 top
Q308  108.9,48.26 0 top
Q309  108.9,41.91 0 top
Q310  108.9,35.56 0 top
Q311  108.9,29.21 0 top
QG101  25.08,35.88 270 top
R101  24.77,62.87 180 top
R102  24.77,65.72 180 top
R103  24.77,68.58 180 top
R104  24.77,71.44 180 top
R105  24.77,74.3 180 top
R106  40.64,81.28 0 top
R107  40.64,84.14 180 top
R108  24.77,48.26 180 top
R109  24.77,57.15 0 top
R201  52.39,19.37 270 top
R202  55.24,19.37 270 top
R301  99.06,94.61 180 top
R302  99.06,88.27 180 top
R303  99.06,81.92 180 top
R304  99.06,75.56 180 top
R305  99.06,69.22 180 top
R306  99.06,62.87 180 top
R307  99.06,56.52 180 top
R308  99.06,50.16 180 top
R309  99.06,43.81 180 top
R310  99.06,37.47 180 top
R311  99.06,31.11 180 top
RN301  68.26,86.04 270 top
RN302  68.26,64.77 270 top
RN303  68.26,43.5 270 top
SV101  60.96,8.26 180 top
V101  24.77,86.36 180 top
X101  5.08,10.48 270 top
X102  5.08,30.48 270 top
X201  94.3,11.11 180 top
X301  130.18,53.02 0 top
X302  130.18,28.89 0 top
X303  130.18,40.96 0 top
X304  133.67,79.38 0 top

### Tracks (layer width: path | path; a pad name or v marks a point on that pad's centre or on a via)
1-WIRE
  Top 0.61: IC102.2 35.56,87.31 37.47,85.41 37.47,78.11 35.88,76.52 IC101.1
+5V  (via drill 0.5)
  Top 0.406: IC201.9 73.66,48.9 78.74,43.81 IC201.18
  Top 0.813: 31.43,53.66 31.43,63.5 30.48,64.45 v18.41,64.45 16.51,66.36 v16.51,76.52 v16.51,77.79 v16.51,79.06 v16.51,80.33 | IC101.10 31.43,53.66 | QG101.14 31.43,46.04 31.43,53.66 | 50.8,4.45 50.8,14.29 | 50.8,14.29 50.8,14.61 49.53,15.88 IC104.18 | 50.8,4.45 IC103.8 | 50.8,4.45 62.55,4.45 63.5,5.4 SV101.2 65.41,8.89 65.41,11.75 62.23,14.92 DC201.2 62.23,21.91 C202.1 v61.28,48.58 | R202.2 R201.2 50.8,14.29 | LED212.A 90.17,22.54 88.27,20.64 85.72,20.64 84.45,19.37 84.45,8.57 85.41,7.62 X201.3-1 | LED201.A LED202.A LED203.A LED204.A LED205.A LED206.A LED207.A LED208.A LED209.A LED210.A LED211.A LED212.A | LED212.A 90.17,44.77
  Bottom 0.61: R103.2 R102.2 19.68,65.09 19.05,64.45 v18.41,64.45
  Bottom 0.813: IC104.18 IC104.17 45.72,15.24 43.18,12.7 IC103.3 | 29.21,18.73 29.21,25.4 30.8,26.99 30.8,40.01 28.89,41.91 QG101.14 | 29.21,18.73 29.21,13.34 IC105.3 30.48,10.16 31.11,9.53 33.97,9.53 38.1,5.4 38.1,3.49 39.37,2.22 46.04,2.22 46.99,3.17 46.99,4.13 47.31,4.45 IC103.8 IC103.7 | IC101.10 45.09,53.66 46.35,54.93 50.48,54.93 51.12,54.29 51.12,51.75 50.48,51.12 IC101.30 | 33.02,89.53 26.04,89.53 22.23,85.72 V101.OUT 18.1,83.82 16.51,82.23 v16.51,80.33 v16.51,79.06 v16.51,77.79 v16.51,76.52 | v18.41,64.45 18.41,62.87 | 18.41,62.87 18.41,58.42 R109.1 | R101.2 18.41,62.87 | C103.+ 43.81,92.08 C107.1 40.96,91.12 39.37,89.53 33.02,89.53 | 33.02,87.95 IC102.3 33.02,89.53 | IC201.9 71.44,48.9 71.12,48.58 v61.28,48.58 | C106.1 25.72,17.14 27.3,18.73 29.21,18.73
  Bottom 1.016: SV101.2 77.15,6.99 77.79,7.62 X201.3-1 X201.2-1 X201.1-1
+18V  (via drill 0.5)
  Top 0.406: R106.1 35.56,81.6 34.29,82.87 34.29,85.41 33.66,86.04 32.38,86.04 31.75,86.68 31.75,90.49 32.38,91.12 34.29,91.12 36.51,93.34 D103.C
  Top 1.27: D102.A 18.1,87.95 v17.78,87.63 v16.83,86.68 v15.88,85.72 12.06,81.92 4.45,81.92 3.17,80.64 3.17,69.22 14.92,57.47 v14.92,32.07 14.92,13.34 13.65,12.06 9.46,12.06 X101.6
  Bottom 1.27: X102.6 14.86,32 v14.92,32.07 | D103.C 36.2,93.34 33.97,91.12 24.77,91.12 21.59,87.95 D102.A 18.1,87.95 v17.78,87.63 v16.83,86.68 v15.88,85.72
/CS-MBC  (via drill 0.5)
  Top 0.406: v39.37,66.36 39.37,26.35 40.01,25.72 v41.91,25.72
  Bottom 0.406: v39.37,66.36 IC101.5 32.7,66.36 30.48,68.58 R103.1 | v41.91,25.72 41.91,20.64 43.18,19.37 IC104.16
/CS-MEM  (via drill 0.5)
  Top 0.406: v46.67,71.44 v46.67,65.09 46.67,25.08 46.99,24.77 v46.99,20.95 | v46.99,17.78 46.99,14.29 48.26,13.02 IC103.1
  Bottom 0.406: IC101.38 v46.67,71.44 | v46.99,20.95 v46.99,17.78 | R102.1 31.43,65.72 32.07,65.09 v46.67,65.09
/INT  (via drill 0.5)
  Top 0.406: IC101.3 32.38,71.44 31.11,70.17 v28.26,70.17 | v27.62,26.99 29.21,25.4 29.21,22.23 v30.48,20.95
  Bottom 0.406: v28.26,70.17 27.62,69.53 27.62,55.88 26.67,54.93 26.67,27.94 v27.62,26.99 | v30.48,20.95 30.48,19.68 33.02,17.14 IC104.12
/RES  (via drill 0.5)
  Top 0.406: v33.02,26.35 34.61,26.35 35.56,27.3 35.56,56.2 | IC101.9 35.56,56.2 | 35.56,56.2 v35.56,60.01 35.56,67.94 v36.51,68.9 | R101.1 v29.84,60.01 C102.1
  Bottom 0.406: v33.02,26.35 31.75,25.08 31.75,20.95 34.29,18.41 34.29,10.48 37.47,7.3 40.96,7.3 42.86,9.21 58.1,9.21 SV101.5 | v36.51,68.9 IC101.37 | v29.84,60.01 v35.56,60.01
AREF
  Bottom 0.406: IC101.32 C101.1
CAN-H  (via drill 0.5)
  Top 0.406: v25.4,53.98 OK101.4 | IC105.7 33.02,7.3 32.07,8.26 v23.81,8.26 | v11.11,33.97 v11.11,13.97
  Bottom 0.406: v25.4,53.98 25.4,34.92 24.51,34.04 X102.8 11.05,34.04 v11.11,33.97 | v23.81,8.26 23.81,13.34 23.18,13.97 v11.11,13.97 9.46,13.97 X101.8
CAN-L  (via drill 0.5)
  Top 0.406: v12.7,35.56 v12.7,15.24
  Bottom 0.406: R108.2 24.13,43.81 24.13,36.51 23.18,35.56 v12.7,35.56 8.89,35.56 7.62,34.29 X102.7 | X101.7 7.62,14.29 8.57,15.24 v12.7,15.24 24.45,15.24 25.08,14.61 25.08,7.62 25.72,6.99 29.84,6.99 30.48,6.35 IC105.6
GND  (via drill 0.5)
  Top 0.406: OK202.13 58.42,63.5 58.74,63.18 | 58.74,68.58 OK202.11 | OK202.9 58.74,73.66 | OK201.15 58.74,79.69 | OK201.13 58.74,84.77 | OK201.11 58.74,89.85 | OK202.15 58.74,58.42 | OK101.2 17.46,51.44 17.14,51.75 | v58.74,52.39 OK203.9 | OK203.11 58.74,47.31 | 58.74,41.91 58.42,42.23 OK203.13
  Top 0.61: SV101.6 58.1,6.99 56.83,8.26 56.83,14.92 58.1,16.19 DC201.1
  Top 0.813: IC101.31 C101.2 | 24.77,86.68 V101.GND | 24.77,86.68 28.26,86.68 30.16,84.77 v30.16,83.5 v30.16,82.23 v31.11,81.28 C104.2 | D101.K 11.43,77.15 20.95,86.68 24.77,86.68 | 51.75,92.39 51.44,92.08 50.8,92.08 | DC201.1 59.69,20.64 58.74,21.59 C202.2 58.74,41.91 58.74,47.31 v58.74,52.39 v58.74,53.66 v58.74,54.93 58.74,58.42 58.74,63.18 58.74,68.58 58.74,73.66 58.74,79.69 58.74,84.77 58.74,89.85 58.74,93.98 57.78,94.93 OK201.9 54.29,94.93 51.75,92.39 | 9.59,10.16 X101.4 | IC201.10 73.03,46.35 78.11,41.27 IC201.17 IC201.16 IC201.15 80.96,36.2 82.23,34.92 82.23,13.65 v81.6,13.65 | v81.6,13.65 v80.33,13.65 | v81.6,13.65 v82.87,13.65 | 51.75,89.53 51.75,83.82 C105.- v50.48,82.55 v49.53,81.6 v48.26,81.6 | 51.75,89.53 51.75,91.95 | 51.75,91.95 C103.- | 51.75,89.53 45.4,89.53 44.45,88.58 C107.2 42.55,88.27 IC102.1 | 51.75,91.95 51.75,92.39 | C106.2 16.51,17.14
  Top 1.016: QG101.7 21.27,27.62 16.51,22.86 v16.51,22.38 16.51,17.14 16.51,11.43 16.19,11.11 | 16.19,11.11 14.92,9.53 | 14.92,9.53 33.02,9.53 | 33.02,9.53 IC105.2 | IC105.8 35.56,9.53 | 35.56,9.53 33.02,9.53 | 35.56,9.53 38.1,9.53 IC103.4 | X101.S@2 11.27,2.38 14.92,6.03 14.92,9.53 | 14.92,9.53 14.92,9.84 15.24,10.16 | 16.19,11.11 15.24,10.16 | 15.24,10.16 9.59,10.16 | X101.5 7.75,10.99 X101.4
  Top 1.27: v5.4,71.44 v8.26,68.58 16.83,60.01 17.14,60.01 | IC104.9 23.18,28.26 QG101.7 18.73,28.26 v18.1,28.89 v18.1,38.58 18.1,44.77 17.14,45.72 17.14,51.75 17.14,60.01 | C102.2 17.14,60.01
  Bottom 0.61: C104.2 R107.2
  Bottom 0.813: IC101.11 44.13,51.12 46.67,53.66 IC101.31 | C101.2 v58.74,53.66 | v58.74,54.93 v58.74,53.66 | v58.74,53.66 v58.74,52.39 | X102.S@1 v18.1,38.58 | X102.4 7.62,29.97 | 7.62,29.97 X102.5 | 7.62,29.84 7.62,29.97 | X102.3 7.62,29.84 | 7.62,29.84 10.16,29.84 11.11,28.89 v18.1,28.89 | DC201.1 59.69,14.29 60.33,13.65 v80.33,13.65 v81.6,13.65 v82.87,13.65 84.45,13.65 85.41,14.61 | v30.16,83.5 v30.16,82.23 v31.11,81.28 C104.2 32.7,80.33 33.66,79.38 39.05,79.38 42.23,82.55 46.67,82.55 47.62,81.6 v48.26,81.6 v49.53,81.6 v50.48,82.55 C105.-
  Bottom 1.016: X101.S@1 X102.S@2 v16.51,22.38 | 85.41,14.61 X201.3-4 X201.2-4 X201.1-4
  Bottom 1.27: 3.17,77.15 3.17,88.39 5.28,90.49 CON101.2 | 3.17,77.15 D101.K | 3.17,77.15 3.17,73.66 v5.4,71.44 v6.35,70.48 v7.3,69.53 v8.26,68.58
GNDA
  Top 0.813: DC201.3 C201.2
  Top 1.016: DC201.3 64.77,14.61 68.58,10.79 68.58,3.17 70.48,1.27 97.16,1.27 98.42,2.54 98.42,22.54 99.69,23.81 133.35,23.81 134.62,25.08 134.62,30.48 | 134.62,30.48 X302.1 | X303.1 134.62,42.55 | 134.62,42.55 134.62,30.48 | X301.1 133.67,54.61 134.62,53.66 134.62,42.55
I01  (via drill 0.5)
  Top 0.406: v40.32,38.42 40.32,77.15 42.86,79.69 49.53,79.69 53.02,83.19 53.02,90.17 54.93,92.39 OK201.10
  Bottom 0.406: IC101.16 v40.32,38.42
I02  (via drill 0.5)
  Top 0.406: v41.27,35.88 41.27,76.83 43.18,78.74 49.85,78.74 53.98,82.87 53.98,86.36 54.93,87.31 OK201.12
  Bottom 0.406: IC101.17 v41.27,35.88
I03  (via drill 0.5)
  Top 0.406: v42.23,33.34 42.23,76.52 43.5,77.79 50.48,77.79 54.93,82.23 OK201.14
  Bottom 0.406: IC101.18 v42.23,33.34
I04  (via drill 0.5)
  Top 0.406: v43.18,30.8 43.18,73.03 45.4,75.25 51.44,75.25 53.34,77.15 OK201.16
  Bottom 0.406: IC101.19 v43.18,30.8
I05
  Top 0.406: IC101.36 50.48,66.36 51.44,67.31 51.44,70.17 52.39,71.12 OK202.10
I06
  Top 0.406: IC101.35 51.75,63.82 53.98,66.04 OK202.12
I07
  Top 0.406: IC101.34 51.12,61.28 51.44,60.96 OK202.14
I08
  Top 0.406: IC101.33 52.39,58.74 55.24,55.88 OK202.16
I09
  Top 0.406: IC101.29 52.07,48.58 53.34,49.85 OK203.10
I10
  Top 0.406: IC101.28 52.39,46.04 53.66,44.77 OK203.12
I11
  Top 0.406: IC101.27 49.53,43.5 53.34,39.69 OK203.14
IN
  Top 1.422: 119.06,27.94 119.06,26.35 120.02,25.4 127.95,25.4 128.91,26.35 130.18,26.35 X302.2 | 119.06,27.94 119.06,31.43 | 119.06,31.43 119.06,34.29 | 119.06,34.29 119.06,37.47 | 119.06,37.47 119.06,40.64 | 119.06,40.64 119.06,43.5 | 119.06,43.5 119.06,46.99 | 119.06,46.99 119.06,50.16 | 119.06,50.16 119.06,53.66 | 119.06,53.66 119.06,56.2 | 119.06,56.2 119.06,59.69 | 119.06,59.69 119.06,62.87 | 119.06,62.87 119.06,66.04 | 119.06,66.04 119.06,69.22 | 119.06,69.22 119.06,72.39 | 119.06,72.39 119.06,75.56 | 119.06,75.56 119.06,78.74 | 119.06,78.74 119.06,81.92 | 119.06,81.92 119.06,85.09 | 119.06,85.09 119.06,88.27 | 119.06,88.27 119.06,91.44 | 119.06,91.44 119.06,93.98 119.7,94.61 D308.A | D309.A 119.06,88.27 | D310.A 119.06,81.92 | D311.A 119.06,75.56 | D312.A 119.06,69.22 | D313.A 119.06,62.87 | D314.A 119.38,56.52 119.06,56.2 | D326.A 119.06,50.16 | D327.A 119.38,43.81 119.06,43.5 | 119.06,37.47 D328.A 128.59,37.47 X303.2 | D329.A 119.38,31.11 119.06,31.43 | 119.06,27.94 D325.C 111.44,27.94 Q311.1 | 119.06,34.29 D324.C 111.44,34.29 Q310.1 | 119.06,40.64 D323.C 111.44,40.64 Q309.1 | 119.06,46.99 D322.C 111.44,46.99 Q308.1 | 119.06,53.66 118.75,53.34 D307.C 111.44,53.34 Q307.1 | 119.06,59.69 D306.C 111.12,59.69 Q306.1 | 119.06,66.04 D305.C 111.12,66.04 Q305.1 | 119.06,72.39 D304.C 111.12,72.39 Q304.1 | 119.06,78.74 D303.C 111.12,78.74 Q303.1 | 119.06,85.09 D302.C 111.12,85.09 Q302.1 | 119.06,91.44 D301.C 111.12,91.44 Q301.1
LED-G
  Top 0.406: IC101.2 32.7,74.3 R105.1
LED-R
  Bottom 0.61: IC101.4 32.38,68.9 R104.1
MISO  (via drill 0.5)
  Top 0.406: v37.47,61.28 v37.47,27.3 | IC104.15 40.64,15.56 42.23,13.97 45.09,13.97 45.72,13.34 IC103.2 | v63.5,11.43 SV101.1
  Bottom 0.406: IC101.7 v37.47,61.28 | v37.47,27.3 39.37,25.4 39.37,20.64 40.64,19.37 IC104.15 | IC103.2 45.72,10.48 46.04,10.16 49.21,10.16 50.48,11.43 v63.5,11.43
MOSI  (via drill 0.5)
  Top 0.406: v38.42,63.82 38.42,26.67 v36.83,25.08 | IC104.14 38.1,14.61 38.73,13.97 40.96,13.97 41.91,13.02 41.91,6.35 40.64,5.08 IC103.5 40.64,2.54 41.27,1.91 v60.96,1.91
  Bottom 0.406: IC101.6 v38.42,63.82 | v36.83,25.08 36.83,20.64 38.1,19.37 IC104.14 | v60.96,1.91 SV101.4
N$1
  Top 0.406: IC104.1 48.26,20.64 46.35,18.73 35.24,18.73 34.29,17.78 34.29,13.34 IC105.1
N$2
  Top 0.406: IC104.2 45.72,20.64 44.77,19.68 30.16,19.68 29.21,18.73 29.21,13.34 IC105.4
N$4
  Bottom 0.406: OK101.3 28.57,49.53 R108.1
N$6
  Bottom 0.813: C105.+ 45.72,86.68 33.02,86.68 | 33.02,86.68 31.11,86.68 D102.C 28.57,87.95 27.3,86.68 V101.IN | C104.1 32.7,86.36 33.02,86.68
N$7
  Top 0.61: R109.2 24.13,57.15 OK101.1
  Bottom 0.406: 7.56,8.89 X101.3
  Bottom 0.61: OK101.1 15.24,53.98 14.29,53.02 14.29,42.23 13.34,41.27 4.45,41.27 2.54,39.37 2.54,11.11 4.76,8.89 7.56,8.89
N$9
  Bottom 0.406: D101.AR 11.75,74.61 14.92,71.44 R104.2
N$10
  Top 0.61: IC201.1 72.39,70.8 70.8,72.39 70.8,91.44 71.75,92.39 85.41,92.39 LED201.K
N$11
  Top 0.61: IC201.24 84.45,59.05 85.09,58.42 85.09,45.72 87,43.81 LED209.K
N$13
  Bottom 0.406: D101.AG 10.79,79.69 12.7,77.79 12.7,74.93 13.65,73.98 19.37,73.98 R105.2
N$16
  Top 0.61: IC201.21 81.92,51.44 82.23,51.12 82.23,42.86 85.09,40.01 85.09,26.99 LED212.K
N$18
  Top 0.61: IC201.2 73.98,66.67 74.61,67.31 74.61,70.48 72.07,73.03 72.07,87.31 73.03,88.27 LED202.K
N$19
  Top 0.61: IC201.3 73.98,64.14 74.61,64.77 74.61,66.04 75.56,66.99 75.56,71.44 73.34,73.66 73.34,81.28 73.98,81.92 LED203.K
N$22
  Top 0.61: IC201.4 73.98,61.59 74.61,62.23 74.61,63.5 75.56,64.45 75.56,65.72 76.52,66.67 76.52,69.85 82.23,75.56 LED204.K
N$23
  Top 0.61: IC201.5 73.98,59.05 74.61,59.69 74.61,60.96 75.56,61.91 75.56,63.18 76.52,64.14 76.52,65.41 77.47,66.36 77.47,66.99 78.42,67.94 84.14,67.94 85.41,69.22 LED205.K
N$27
  Top 1.27: Q301.2 106.68,96.52 96.52,96.52 94.61,94.61 R301.2
N$32
  Top 0.61: IC201.6 74.93,56.52 75.56,57.15 75.56,60.64 76.52,61.59 76.52,62.87 77.47,63.82 77.47,64.77 78.11,65.41 85.09,65.41 LED206.K
N$33
  Bottom 1.27: Q301.3 105.41,92.71 D315.C
N$34
  Top 0.61: IC201.7 75.56,53.98 76.52,54.93 76.52,60.33 77.47,61.28 77.47,62.55 77.79,62.87 84.45,62.87 87.63,59.69 LED207.K
N$35
  Top 0.61: IC201.8 76.83,51.44 77.47,52.07 77.47,59.69 78.11,60.33 84.77,60.33 86.36,58.74 86.36,51.44 LED208.K
N$36
  Top 0.61: IC201.22 82.55,53.98 83.19,53.34 83.19,43.81 86.36,40.64 86.36,32.38 LED211.K
N$37
  Top 0.61: IC201.23 83.5,56.52 84.14,55.88 84.14,44.77 87.63,41.27 LED210.K
N$38
  Bottom 0.61: RN301.1 75.88,94.93 79.38,91.44 D315.A
N$40
  Top 1.27: Q302.2 107,89.85 96.2,89.85 94.61,88.27 R302.2
N$41
  Bottom 1.27: Q302.3 105.41,86.36 D316.C
N$49
  Bottom 0.61: D316.A 82.55,85.09 77.79,89.85 RN301.3
N$51
  Top 1.27: Q303.2 107,83.5 96.2,83.5 94.61,81.92 R303.2
N$52
  Bottom 1.27: Q303.3 105.41,80.01 D317.C
N$53
  Bottom 0.61: D317.A 85.41,78.74 79.38,84.77 RN301.5
N$55
  Top 1.27: Q304.2 107,77.15 96.2,77.15 94.61,75.56 R304.2
N$56
  Bottom 1.27: Q304.3 105.41,73.66 D318.C
N$57
  Bottom 0.61: D318.A 75.25,72.39 73.34,74.3 73.34,77.47 71.12,79.69 RN301.7
N$59
  Top 1.27: Q305.2 107,70.8 95.89,70.8 94.3,69.22 R305.2
N$60
  Bottom 1.27: Q305.3 105.41,67.31 D319.C
N$61
  Bottom 0.61: D319.A 84.45,66.04 82.55,67.94 78.11,67.94 72.39,73.66 RN302.1
N$63
  Top 1.27: Q306.2 107,64.45 96.2,64.45 94.61,62.87 R306.2
N$66
  Bottom 1.27: Q306.3 105.41,60.96 D320.C
N$67
  Bottom 0.61: D320.A 86.68,59.69 86.04,60.33 77.79,60.33 76.52,61.59 76.52,66.99 75.56,67.94 68.9,67.94 RN302.3
N$69
  Top 1.27: Q307.2 107.31,58.1 96.2,58.1 94.61,56.52 R307.2
N$70
  Bottom 1.27: Q307.3 105.41,54.61 D321.C
N$71
  Bottom 0.61: D321.A 84.14,53.34 82.23,55.24 76.52,55.24 75.56,56.2 75.56,62.23 74.93,62.87 68.9,62.87 RN302.5
N$73
  Top 1.27: Q308.2 107.31,51.75 96.2,51.75 94.61,50.16 R308.2
N$74
  Bottom 1.27: Q308.3 105.41,48.26 D330.C
N$75
  Bottom 0.61: D330.A 83.19,46.99 82.55,47.62 76.83,47.62 75.88,48.58 75.88,52.07 74.61,53.34 74.61,57.15 73.98,57.78 68.9,57.78 RN302.7
N$77
  Top 1.27: Q309.2 107.31,45.4 96.2,45.4 94.61,43.81 R309.2
N$78
  Bottom 1.27: Q309.3 105.41,41.91 D331.C
N$79
  Bottom 0.61: D331.A 83.82,40.64 81.92,42.55 77.47,42.55 76.52,43.5 76.52,46.67 74.93,48.26 74.93,51.75 73.98,52.7 68.58,52.7 RN303.1
N$81
  Top 1.27: Q310.2 107.31,39.05 96.2,39.05 94.61,37.47 R310.2
N$82
  Bottom 1.27: Q310.3 105.41,35.56 D332.C
N$83
  Bottom 0.61: D332.A 76.52,34.29 75.56,35.24 75.56,46.35 74.3,47.62 68.58,47.62 RN303.3
N$85
  Top 1.27: Q311.2 107.31,32.7 96.2,32.7 94.61,31.11 R311.2
N$86
  Bottom 1.27: Q311.3 105.41,29.21 D333.C
N$87
  Bottom 0.61: D333.A 76.83,27.94 74.61,30.16 74.61,41.59 73.66,42.55 68.58,42.55 RN303.5
OUT1
  Top 1.016: X304.1 126.7,94.95 123.51,91.76 123.19,91.76 D301.A
  Bottom 1.27: D301.A 119.38,91.44 116.2,94.61 D308.C 110.81,96.52 106.36,96.52 104.46,94.61 R301.1
OUT2
  Top 1.016: X304.2 126.7,91.45 125.09,89.85 125.09,85.72 124.46,85.09 D302.A
  Bottom 1.27: D302.A 119.7,88.27 D309.C 110.81,90.17 106.68,90.17 104.78,88.27 R302.1
OUT3
  Top 1.016: X304.3 127.96,87.95 127,87 127,80.01 125.73,78.74 D303.A
  Bottom 1.27: D303.A 119.7,81.92 D310.C 110.81,83.82 107,83.82 105.09,81.92 R303.1
OUT4
  Bottom 1.016: X304.4 127.01,84.46 125.09,82.55 125.09,73.66 123.83,72.39 D304.A
  Bottom 1.27: D304.A 119.7,75.56 D311.C 110.81,77.47 106.68,77.47 104.78,75.56 R304.1
OUT5
  Bottom 1.016: X304.5 127.64,80.97 127,80.33 127,68.58 124.46,66.04 D305.A
  Bottom 1.27: D305.A 119.7,69.22 D312.C 110.81,71.12 107,71.12 105.09,69.22 R305.1
OUT6
  Top 1.016: X304.6 127.01,77.48 125.09,75.56 125.09,60.64 124.14,59.69 D306.A
  Bottom 1.27: D306.A 119.7,62.87 D313.C 110.81,64.77 106.68,64.77 104.78,62.87 R306.1
OUT7
  Top 1.016: X304.7 127.95,73.98 127,73.03 127,59.05 125.41,57.47 125.41,54.61 124.14,53.34 D307.A
  Bottom 1.27: D307.A 119.7,56.52 D314.C 110.81,58.42 106.68,58.42 104.78,56.52 R307.1
OUT8
  Top 1.016: X304.8 133.36,70.48 133.99,69.85 133.99,59.69 133.67,59.37 130.18,59.37 127,56.2 127,48.58 125.41,46.99 D322.A
  Bottom 1.27: D322.A 119.7,50.16 D326.C 110.81,52.07 107,52.07 105.09,50.16 R308.1
OUT9
  Bottom 1.016: 119.7,43.81 120.02,43.81 123.19,40.64 124.46,40.64 125.41,41.59 125.41,64.14 128.27,66.99 130.15,66.99 X304.9
  Bottom 1.27: D323.A 119.7,43.81 D327.C 110.81,45.72 107,45.72 105.09,43.81 R309.1
OUT10
  Bottom 1.016: D324.A 125.73,34.29 127,35.56 127,56.2 130.18,59.37 X304.10
  Bottom 1.27: D324.A 119.7,37.47 D328.C 110.81,39.37 107,39.37 105.09,37.47 R310.1
OUT11
  Bottom 1.016: X301.2 134.31,51.11 135.89,49.53 135.89,34.92 134.3,33.34 127.95,33.34 125.73,31.11 125.73,29.21 124.46,27.94 D325.A
  Bottom 1.27: D325.A 119.7,31.11 D329.C 110.81,33.02 107,33.02 105.09,31.11 R311.1
PLUGGED  (via drill 0.5)
  Top 0.406: v17.78,75.25 v17.78,70.17
  Bottom 0.406: CON101.3 10.65,83.33 13.97,80.01 13.97,76.2 14.92,75.25 v17.78,75.25 | v17.78,70.17 25.4,70.17 27.94,72.71 44.77,72.71 46.04,73.98 IC101.39
Q-CLK
  Top 0.406: IC101.13 33.02,46.04 30.8,43.81 30.8,28.26 | 30.8,28.26 30.8,23.81 IC104.8 | 30.8,28.26 QG101.8
S01
  Bottom 0.61: OK201.8 65.09,94.93 67.63,92.39 RN301.2
S02
  Bottom 0.61: OK201.6 65.09,89.85 67.63,87.31 RN301.4
S03
  Bottom 0.61: OK201.4 65.09,84.77 67.63,82.23 RN301.6
S04
  Bottom 0.61: OK201.2 65.09,79.69 67.63,77.15 RN301.8
S05
  Bottom 0.61: OK202.8 65.09,73.66 67.63,71.12 RN302.2
S06
  Bottom 0.61: OK202.6 65.09,68.58 67.63,66.04 RN302.4
S07
  Bottom 0.61: OK202.4 65.09,63.5 67.63,60.96 RN302.6
S08
  Bottom 0.61: OK202.2 65.09,58.42 67.63,55.88 RN302.8
S09
  Bottom 0.61: OK203.8 65.09,52.39 67.63,49.85 RN303.2
S10
  Bottom 0.61: OK203.6 65.09,47.31 67.63,44.77 RN303.4
S11
  Bottom 0.61: OK203.4 65.09,42.23 67.63,39.69 RN303.6
SCK  (via drill 0.5)
  Top 0.406: v36.51,58.74 v36.51,26.35 | v38.1,8.26 38.1,6.99 v39.05,6.03
  Bottom 0.406: IC101.8 v36.51,58.74 | v36.51,26.35 35.56,26.35 34.29,25.08 34.29,20.64 35.56,19.37 IC104.13 35.56,14.92 38.1,12.38 v38.1,8.26 | 43.18,6.35 IC103.6 | v39.05,6.03 39.37,6.35 43.18,6.35 | 43.18,6.35 54.29,6.35 56.2,8.26 59.69,8.26 SV101.3
SCL  (via drill 0.5)
  Top 0.61: IC201.12 74.3,41.27 75.88,39.69 75.88,27.62 73.34,25.08 v73.34,18.73 v73.34,12.06
  Bottom 0.61: v73.34,12.06 83.23,12.11 X201.3-3 X201.2-3 X201.1-3 | v73.34,18.73 53.02,18.73 52.39,19.37 R201.1 52.39,28.89 50.48,30.8 IC101.22
SDA  (via drill 0.5)
  Top 0.61: IC201.13 73.66,38.73 74.61,37.78 74.61,27.94 72.07,25.4 v72.07,20 v72.07,10.16
  Bottom 0.61: v72.07,20 55.88,20 55.24,20.64 R202.1 55.24,28.89 50.8,33.34 IC101.23 | v72.07,10.16 86.35,10.16 | 86.35,10.16 X201.3-2 | 86.35,10.16 88.97,10.16 X201.2-2 X201.1-2
SPG
  Top 0.61: R106.2 R107.1
  Bottom 0.61: IC101.40 47.94,76.52 45.72,78.74 R106.2
V+
  Top 0.813: 62.55,87.31 62.55,90.49 OK201.7 | 62.55,87.31 62.55,82.23 | 62.55,82.23 62.55,77.15 | 62.55,77.15 62.55,71.12 | 62.55,71.12 62.55,66.04 | 62.55,66.04 62.55,60.96 | 62.55,60.96 62.55,55.88 | 62.55,66.04 OK202.5 | 62.55,77.15 OK201.1 | 62.55,55.88 OK202.1 | DC201.4 C201.1 67.31,23.81 66.36,24.77 63.82,24.77 62.55,26.04 62.55,39.69 | OK201.5 62.55,87.31 | OK201.3 62.55,82.23 | OK202.7 62.55,71.12 | OK202.3 62.55,60.96 | 62.55,39.69 62.55,44.77 | 62.55,44.77 62.55,49.85 | 62.55,49.85 62.55,55.88 | OK203.7 62.55,49.85 | OK203.5 62.55,44.77 | OK203.3 62.55,39.69
V-NETZTEIL1
  Bottom 1.27: D103.A 23.5,93.34 21.27,91.12 14.29,91.12 CON101.1

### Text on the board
Bottom: MBCAN-Projekt | (c) Dr.-Ing. Th. Wiesner | 31.07.2022 | (c) Christian Laguigner | mbc85.brd | bottom
tNames: HW: 22.07.31 | 1 | 1 | 2 | 2 | 3 | +18V | DC | 4 | 3 | 5 | 6 | 4 | (c) Christian Laguigner | (c) Dr.-Ing. Th. Wiesner | MBCAN-Projekt | 7 | RM Gleise | 8 | 5 | 9 | 6 | 10 | 7 | 0 | 8 | B | RM Bühne | 9 | 0 | IN | Bühne | B | 10 | 0 | Bühne | B | Booster | STAND | OUT | mbc-85 | I2C-Bus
